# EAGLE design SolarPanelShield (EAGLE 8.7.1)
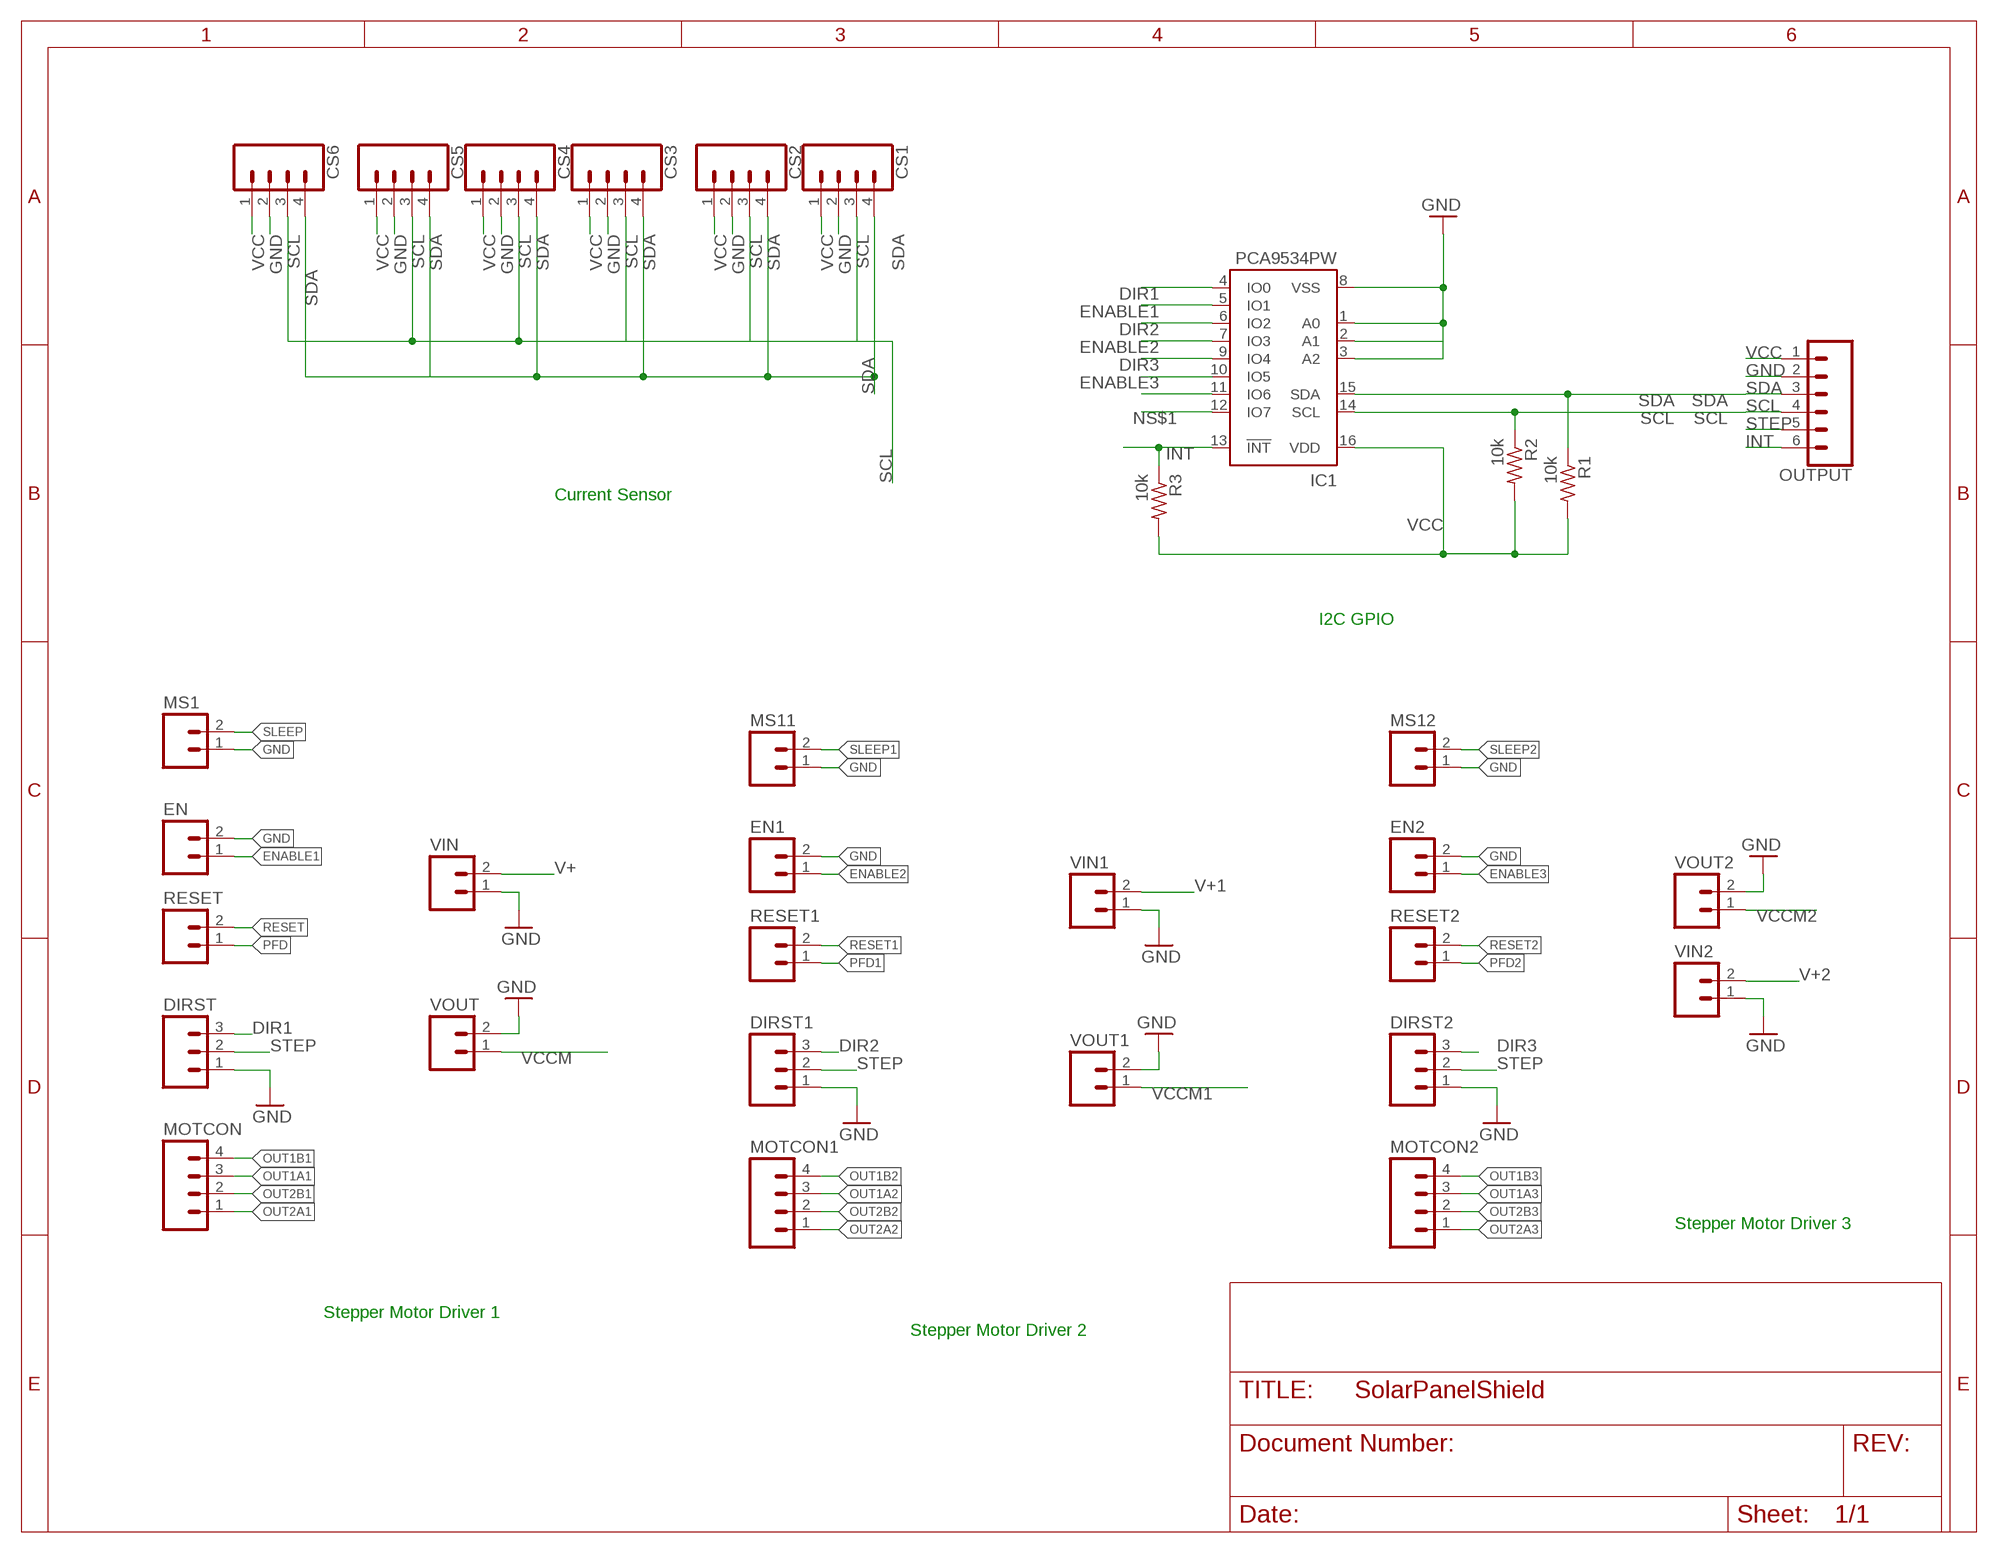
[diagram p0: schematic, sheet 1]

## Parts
CS1  CONN_04LOCK  [1X04_LOCK]
CS2  CONN_04LOCK  [1X04_LOCK]
CS3  CONN_04LOCK  [1X04_LOCK]
CS4  CONN_04LOCK  [1X04_LOCK]
CS5  CONN_04LOCK  [1X04_LOCK]
CS6  CONN_04LOCK  [1X04_LOCK]
DIRST  M031X03_NO_SILK  [1X03_NO_SILK]
DIRST1  M031X03_NO_SILK  [1X03_NO_SILK]
DIRST2  M031X03_NO_SILK  [1X03_NO_SILK]
EN  M021X02_NO_SILK  [1X02_NO_SILK]
EN1  M021X02_NO_SILK  [1X02_NO_SILK]
EN2  M021X02_NO_SILK  [1X02_NO_SILK]
IC1  PCA9534PW  [TSSOP16]
MOTCON  M041X04_NO_SILK  [1X04_NO_SILK]
MOTCON1  M041X04_NO_SILK  [1X04_NO_SILK]
MOTCON2  M041X04_NO_SILK  [1X04_NO_SILK]
MS1  M021X02_NO_SILK  [1X02_NO_SILK]
MS11  M021X02_NO_SILK  [1X02_NO_SILK]
MS12  M021X02_NO_SILK  [1X02_NO_SILK]
OUTPUT  CONN_06SILK_FEMALE_PTH  [1X06]
R1  10k  R-US_R0603  [R0603]
R2  10k  R-US_R0603  [R0603]
R3  10k  R-US_R0603  [R0603]
RESET  M021X02_NO_SILK  [1X02_NO_SILK]
RESET1  M021X02_NO_SILK  [1X02_NO_SILK]
RESET2  M021X02_NO_SILK  [1X02_NO_SILK]
VIN  M021X02_NO_SILK  [1X02_NO_SILK]
VIN1  M021X02_NO_SILK  [1X02_NO_SILK]
VIN2  M021X02_NO_SILK  [1X02_NO_SILK]
VOUT  M021X02_NO_SILK  [1X02_NO_SILK]
VOUT1  M021X02_NO_SILK  [1X02_NO_SILK]
VOUT2  M021X02_NO_SILK  [1X02_NO_SILK]

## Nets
DIR1: DIRST.3 IC1.4(IO0)
DIR2: DIRST1.3 IC1.6(IO2)
DIR3: DIRST2.3 IC1.9(IO4)
ENABLE1: EN.1 IC1.5(IO1)
ENABLE2: EN1.1 IC1.7(IO3)
ENABLE3: EN2.1 IC1.10(IO5)
GND: CS1.2 CS2.2 CS3.2 CS4.2 CS5.2 CS6.2 DIRST1.1 DIRST2.1 DIRST.1 EN1.2 EN2.2 EN.2 IC1.1(A0) IC1.3(A2) IC1.8(VSS) MS1.1 MS11.1 MS12.1 OUTPUT.2 VIN1.1 VIN2.1 VIN.1 VOUT1.2 VOUT2.2 VOUT.2
INT: IC1.13(!INT) OUTPUT.6 R3.1
N$4: IC1.11(IO6)
N$13: IC1.2(A1)
NS$1: IC1.12(IO7)
OUT1A1: MOTCON.3
OUT1A2: MOTCON1.3
OUT1A3: MOTCON2.3
OUT1B1: MOTCON.4
OUT1B2: MOTCON1.4
OUT1B3: MOTCON2.4
OUT2A1: MOTCON.1
OUT2A2: MOTCON1.1
OUT2A3: MOTCON2.1
OUT2B1: MOTCON.2
OUT2B2: MOTCON1.2
OUT2B3: MOTCON2.2
PFD: RESET.1
PFD1: RESET1.1
PFD2: RESET2.1
RESET: RESET.2
RESET1: RESET1.2
RESET2: RESET2.2
SCL: CS1.3 CS2.3 CS3.3 CS4.3 CS5.3 CS6.3 IC1.14(SCL) OUTPUT.4 R2.1
SDA: CS1.4 CS2.4 CS3.4 CS4.4 CS5.4 CS6.4 IC1.15(SDA) OUTPUT.3 R1.1
SLEEP: MS1.2
SLEEP1: MS11.2
SLEEP2: MS12.2
STEP: DIRST1.2 DIRST2.2 DIRST.2 OUTPUT.5
V+: VIN.2
V+1: VIN1.2
V+2: VIN2.2
VCC: CS1.1 CS2.1 CS3.1 CS4.1 CS5.1 CS6.1 IC1.16(VDD) OUTPUT.1 R1.2 R2.2 R3.2
VCCM: VOUT.1
VCCM1: VOUT1.1
VCCM2: VOUT2.1

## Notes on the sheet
- Current Sensor
- I2C GPIO
- Stepper Motor Driver 3
- Stepper Motor Driver 1
- Stepper Motor Driver 2

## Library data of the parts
CS1-CS6 = SparkFun-Connectors:CONN_04: Multi connection point. Often used as Generic Header-pin footprint for 0.1 inch spaced/style header connections On any of the 0.1 inch spaced packages, you can populate with these: Break Away Headers - Straight (PRT-00116) Break Away Male Headers - Right Angle (PRT-00553) Female Headers (PRT-00115)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; PROD_ID: CONN-09696
DIRST DIRST1 DIRST2 = SparkFun:M03: Header 3 Standard 3-pin 0.1" header. Use with straight break away headers (SKU : PRT-00116), right angle break away headers (PRT-00553), swiss pins (PRT-00743), machine pins (PRT-00117), and female headers (PRT-00115). Molex polarized connector foot print use with SKU : PRT-08232 with associated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
EN EN1 EN2 MS1 MS11 MS12 RESET RESET1 RESET2 VIN VIN1 VIN2 VOUT VOUT1 VOUT2 = SparkFun:M02: Header 2
IC1 = micro-philips:PCA9534: 8-bit I2C-bus and SMBus low power I/O port with interrupt Source: www.nxp.com .. PCA9534_3.pdf; MPN: PCA9534PW; OC_FARNELL: 1408285; OC_NEWARK: 18M7516
MOTCON MOTCON1 MOTCON2 = SparkFun:M04: Header 4 Standard 4-pin 0.1" header. Use with straight break away headers (SKU : PRT-00116), right angle break away headers (PRT-00553), swiss pins (PRT-00743), machine pins (PRT-00117), and female headers (PRT-00115). Molex polarized connector foot print use with SKU : PRT-08231 with associated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
OUTPUT = SparkFun-Connectors:CONN_06: Multi connection point. Often used as Generic Header-pin footprint for 0.1 inch spaced/style header connections On any of the 0.1 inch spaced packages, you can populate with these: Break Away Headers - Straight (PRT-00116) Break Away Male Headers - Right Angle (PRT-00553) Female Headers (PRT-00115)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; PROD_ID: CONN-08437
R1-R3 = audio amplifier example:R-US_: RESISTOR, American symbol

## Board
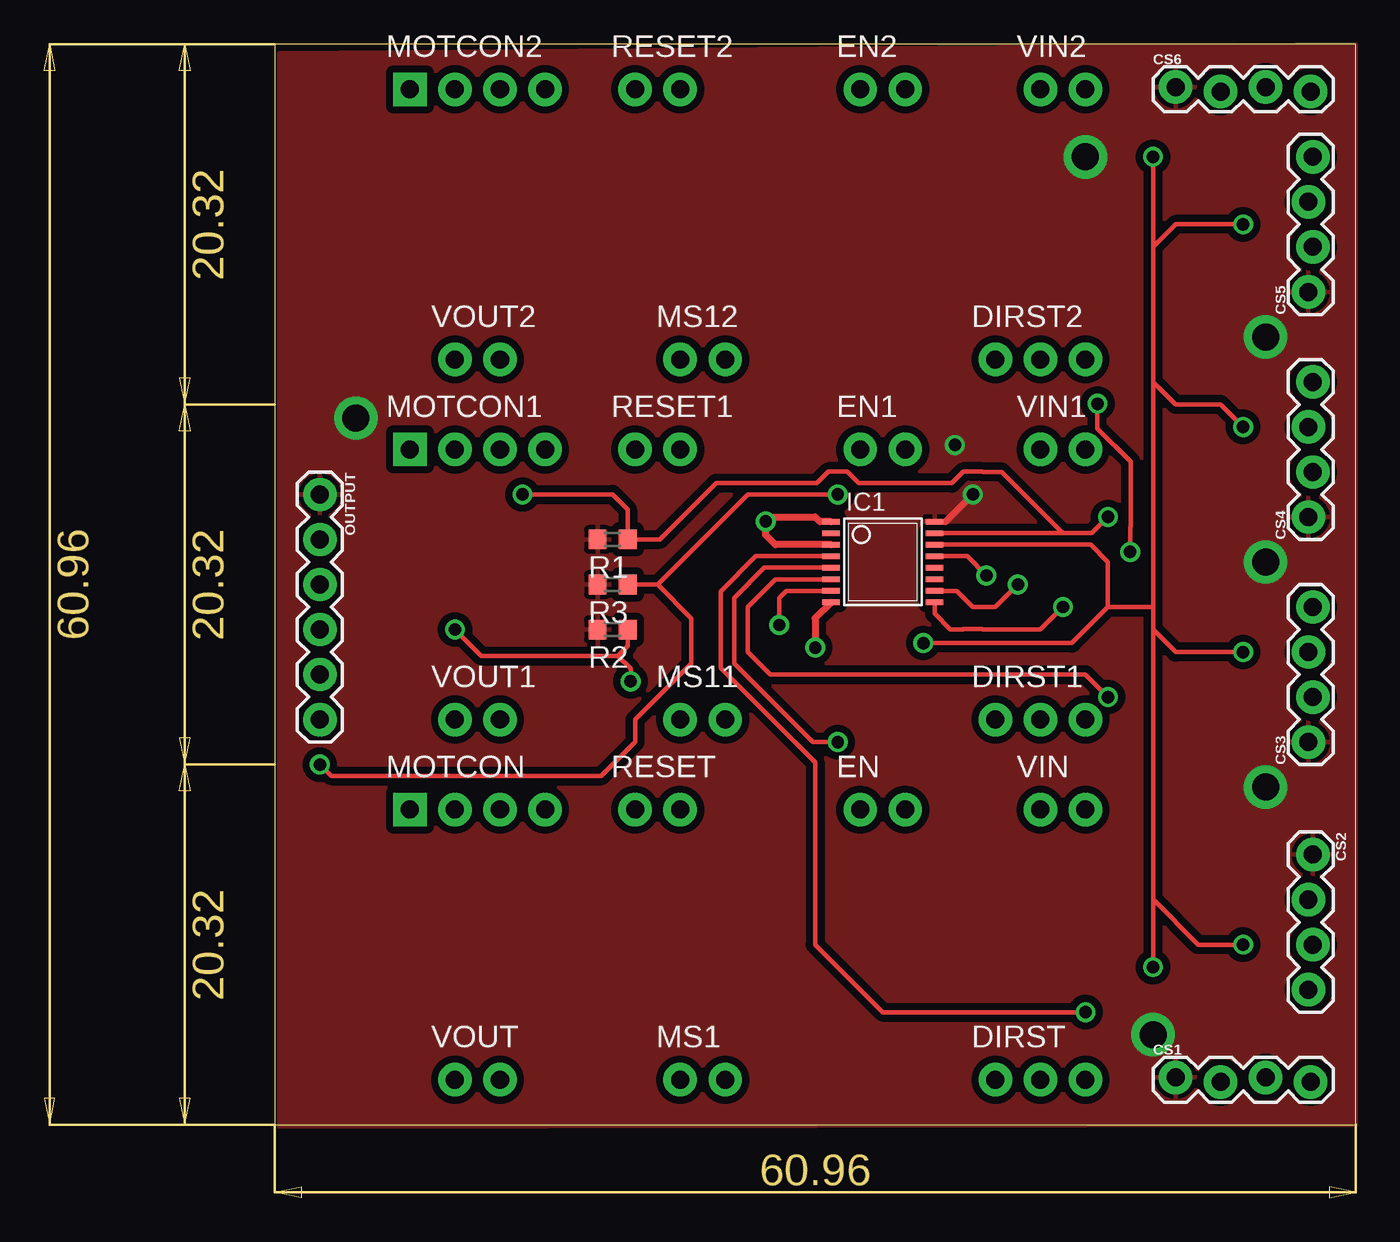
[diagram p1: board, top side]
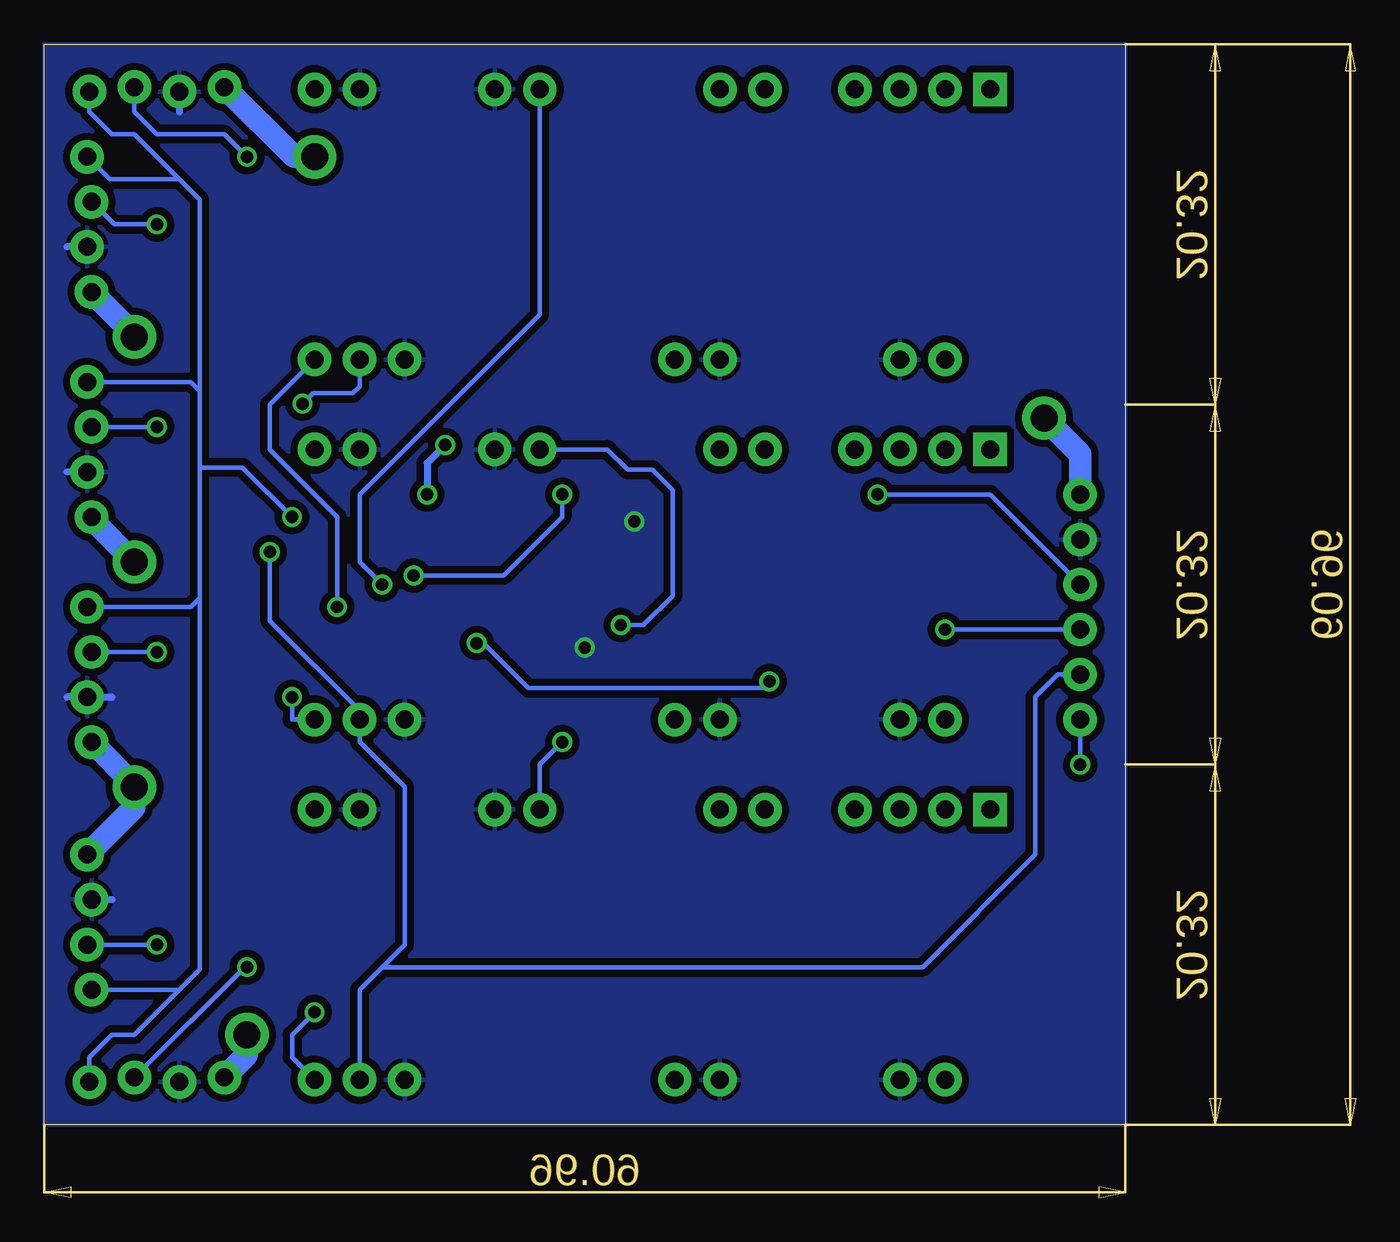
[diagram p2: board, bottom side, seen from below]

Size 73.96 x 65.07 mm. Coordinates in mm from the lower left corner, seen from the top.
Outline: 13,4.11 73.96,4.11 73.96,65.07 13,65.07 13,4.11
Copper layers (1*16): Top 0.035mm / dielectric 1.5mm / Bottom 0.035mm
Design rules "Voltera_DRC": minimum track width 10mil, minimum drill 0.6mm, track to track 10mil, track to pad 10mil, pad to pad 0.6mm, via to via 0.6mm, smd to smd 0mil, copper to edge 0mil, drill to drill 0.8mm, minimum pad ring 0.2mm, minimum via ring 0.2mm, stop-mask expansion 4mil, vias tented up to drill 0mil, thermal gap 10mil

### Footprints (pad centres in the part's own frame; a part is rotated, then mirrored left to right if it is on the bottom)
1X04_LOCK = drill 1.016 pad 1.88: 1 0,0.127; 2 2.54,-0.127; 3 5.08,0.127; 4 7.62,-0.127
1X03_NO_SILK = drill 1.016 pad 1.88: 1 0,0; 2 2.54,0; 3 5.08,0
1X02_NO_SILK = drill 1.016 pad 1.88: 1 0,0; 2 2.54,0
TSSOP16 = smd 0.305 x 0.991: 1 -2.275,-2.918; 2 -1.625,-2.918; 3 -0.975,-2.918; 4 -0.325,-2.918; 5 0.325,-2.918; 6 0.975,-2.918; 7 1.625,-2.918; 8 2.275,-2.918; 9 2.275,2.918; 10 1.625,2.918; 11 0.975,2.918; 12 0.325,2.918; 13 -0.325,2.918; 14 -0.975,2.918; 15 -1.625,2.918; 16 -2.275,2.918
1X04_NO_SILK = drill 1.016 pad 1.88 square: 1 0,0 | drill 1.016 pad 1.88: 2 2.54,0; 3 5.08,0; 4 7.62,0
1X06 = drill 1.016 pad 1.88: 1 0,0; 2 2.54,0; 3 5.08,0; 4 7.62,0; 5 10.16,0; 6 12.7,0
R0603 = smd 1 x 1.1: 1 -0.85,0; 2 0.85,0

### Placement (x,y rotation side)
CS1  63.8,6.65 0 top
CS2  71.42,19.35 270 top
CS3  71.42,25.7 90 top
CS4  71.42,38.4 90 top
CS5  71.42,51.1 90 top
CS6  63.8,62.53 0 top
DIRST  53.64,6.65 0 top
DIRST1  53.64,26.97 0 top
DIRST2  53.64,47.29 0 top
EN  46.02,21.89 0 top
EN1  46.02,42.21 0 top
EN2  46.02,62.53 0 top
IC1  47.29,35.86 270 top
MOTCON  20.62,21.89 0 top
MOTCON1  20.62,42.21 0 top
MOTCON2  20.62,62.53 0 top
MS1  35.86,6.65 0 top
MS11  35.86,26.97 0 top
MS12  35.86,47.29 0 top
OUTPUT  15.54,39.67 270 top
R1  32.05,37.13 180 top
R2  32.05,32.05 180 top
R3  32.05,34.59 180 top
RESET  33.32,21.89 0 top
RESET1  33.32,42.21 0 top
RESET2  33.32,62.53 0 top
VIN  56.18,21.89 0 top
VIN1  56.18,42.21 0 top
VIN2  56.18,62.53 0 top
VOUT  23.16,6.65 0 top
VOUT1  23.16,26.97 0 top
VOUT2  23.16,47.29 0 top

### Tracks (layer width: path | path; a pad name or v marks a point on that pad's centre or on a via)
DIR1  (via drill 0.7)
  Top 0.254: v58.72,10.46 47.29,10.46 43.48,14.27 43.48,24.56 38.15,29.89 38.15,34.21 40.12,36.19 IC1.4
  Bottom 0.254: v58.72,10.46 59.99,9.19 59.99,7.92 DIRST.3
DIR2  (via drill 0.7)
  Top 0.254: IC1.6 41.23,34.88 39.67,33.32 39.67,30.78 40.94,29.51 58.72,29.51 v59.99,28.24
  Bottom 0.254: v59.99,28.24 59.99,26.97 DIRST1.3
DIR3  (via drill 0.7)
  Top 0.254: IC1.9 50.21,32.94 51.1,32.05 51.82,32.05 51.84,32.07 52.9,32.07 52.92,32.05 56.18,32.05 v57.45,33.32
  Bottom 0.254: DIRST2.3 61.26,44.75 61.26,42.21 60.24,41.19 59.99,40.94 57.45,38.4 v57.45,33.32
ENABLE1  (via drill 0.7)
  Top 0.254: IC1.5 40.61,35.54 38.91,33.83 38.91,30.14 43.35,25.7 v44.75,25.7
  Bottom 0.254: v44.75,25.7 46.02,24.43 EN.1
ENABLE2  (via drill 0.7)
  Top 0.254: IC1.7 41.86,34.23 41.45,33.83 v41.45,32.3
  Bottom 0.254: EN1.1 42.21,42.21 41.07,41.07 39.67,41.07 38.53,39.92 38.53,33.95 40.18,32.3 v41.45,32.3
ENABLE3  (via drill 0.7)
  Top 0.254: v54.91,34.59 53.64,33.32 52.37,33.32 51.45,34.23 IC1.10
  Bottom 0.254: v54.91,34.59 56.18,35.86 56.18,39.67 46.02,49.83 EN2.1
GND  (via drill 0.7)
  Top 0.406: IC1.3 41.23,36.84 40.69,37.38 v40.69,38.15 40.94,38.4 43.48,38.4 43.75,38.13 IC1.1 | IC1.8 43.48,32.69 v43.48,31.03
  Bottom 0.406: CS6.2 66.34,61.26 | CS5.2 72.69,53.64 | CS4.2 72.69,40.94 | 70.15,28.24 CS3.2 72.69,28.24 | CS2.2 70.15,16.81
  pour Bottom (isolate 0.406): 26.97,4.11 73.96,4.11 73.96,65.07 13,65.07 13,4.11
INT  (via drill 0.7)
  Top 0.254: IC1.13 52.05,36.19 v53.13,35.1 | v44.75,39.67 39.67,39.67 34.59,34.59 | 34.59,34.59 R3.1 | v15.54,24.43 16.18,23.79 31.41,23.79 33.32,25.7 33.32,26.97 36.5,30.14 36.5,32.69 34.59,34.59
  Bottom 0.254: OUTPUT.6 v15.54,24.43 | v44.75,39.67 44.75,38.4 48.05,35.1 v53.13,35.1
SCL  (via drill 0.7)
  Top 0.254: v62.53,13 62.53,16.81 | 62.53,16.81 62.53,32.05 | 62.53,32.05 62.53,33.32 | 62.53,33.32 62.53,46.02 | 62.53,46.02 62.53,53.64 | 62.53,53.64 v62.53,58.72 | v67.61,14.27 65.07,14.27 62.53,16.81 | v67.61,30.78 63.8,30.78 62.53,32.05 | v67.61,43.48 66.34,44.75 63.8,44.75 62.53,46.02 | v67.61,54.91 63.8,54.91 62.53,53.64 | 59.99,33.32 62.53,33.32 | v23.16,32.05 24.64,30.57 32.35,30.57 | 59.99,33.32 59.99,35.86 59.02,36.84 IC1.14 | 59.99,33.32 57.96,31.29 v49.58,31.29 | R2.1 32.9,31.12 32.35,30.57 | 32.35,30.57 33.07,29.85 v33.07,29.13
  Bottom 0.254: v62.53,13 62.66,13 CS1.3 | v62.53,58.72 63.8,59.99 67.61,59.99 68.88,61.26 CS6.3 | CS2.3 v67.61,14.27 | CS3.3 v67.61,30.78 | CS4.3 v67.61,43.48 | CS5.3 70.02,54.91 v67.61,54.91 | v23.16,32.05 OUTPUT.4 | v49.58,31.29 49.2,31.29 46.66,28.75 33.45,28.75 v33.07,29.13
SDA  (via drill 0.7)
  Top 0.254: IC1.15 57.45,37.48 | 57.45,37.48 59.08,37.48 v59.99,38.4 | v26.97,39.67 32.05,39.67 32.9,38.82 R1.1 34.72,37.13 37.89,40.3 43.56,40.3 44.22,40.96 45.28,40.96 45.94,40.3 51.19,40.3 51.84,40.96 52.9,40.96 52.92,40.94 53.99,40.94 57.45,37.48
  Bottom 0.254: 66.34,57.45 68.88,59.99 70.15,59.99 71.42,61.26 CS6.4 | CS5.4 70.28,57.45 66.34,57.45 | 66.34,11.73 68.88,9.19 70.15,9.19 71.42,7.92 CS1.4 | CS2.4 66.34,11.73 | OUTPUT.3 20.62,39.67 v26.97,39.67 | 66.34,11.73 65.2,12.87 65.2,33.83 | 66.34,57.45 65.2,56.31 65.2,45.51 | 65.2,33.83 65.2,41.19 | 65.2,41.19 65.2,45.51 | 65.2,45.51 65.7,46.02 CS4.4 | 65.2,33.83 65.7,33.32 CS3.4 | 65.2,41.19 62.78,41.19 v59.99,38.4
STEP  (via drill 0.7)
  Top 0.254: v59.4,44.79 59.4,43.4 61.28,41.52 61.28,37.87 61.24,37.83 v61.24,36.43
  Bottom 0.254: DIRST.2 56.18,11.73 54.91,13 | 54.91,13 53.64,14.27 53.64,23.16 56.18,25.7 DIRST1.2 56.18,27.48 61.24,32.54 v61.24,36.43 | 54.91,13 24.43,13 18.08,19.35 18.08,28.24 16.81,29.51 OUTPUT.5 | v59.4,44.79 58.8,45.38 56.56,45.38 56.18,45.77 DIRST2.2
VCC  (via drill 0.7, 1.52)
  Top 0.254: IC1.16 50.84,38.13
  Top 0.406: 50.84,38.13 v52.37,39.67
  Bottom 0.406: v51.35,42.46 52.37,41.45 v52.37,39.67
  Bottom 1.27: CS6.1 59.86,58.72 v58.72,58.72 | CS5.1 68.88,48.69 v68.88,48.56 | CS4.1 71.29,38.27 v68.88,35.86 | CS3.1 68.88,23.29 v68.88,23.16 68.88,22.02 CS2.1 | CS1.1 62.53,8.05 v62.53,9.19 | OUTPUT.1 15.54,41.96 v17.57,43.99
  pour Top (isolate 0.406): 73.96,4.11 13.25,3.98 13.25,64.56 73.96,65.07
